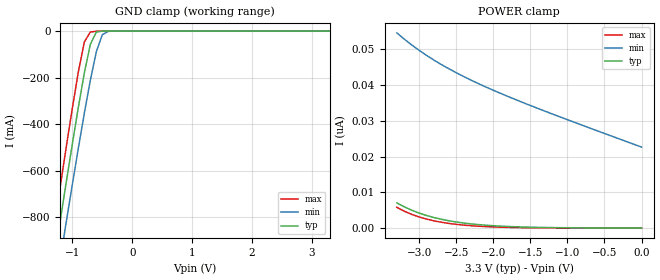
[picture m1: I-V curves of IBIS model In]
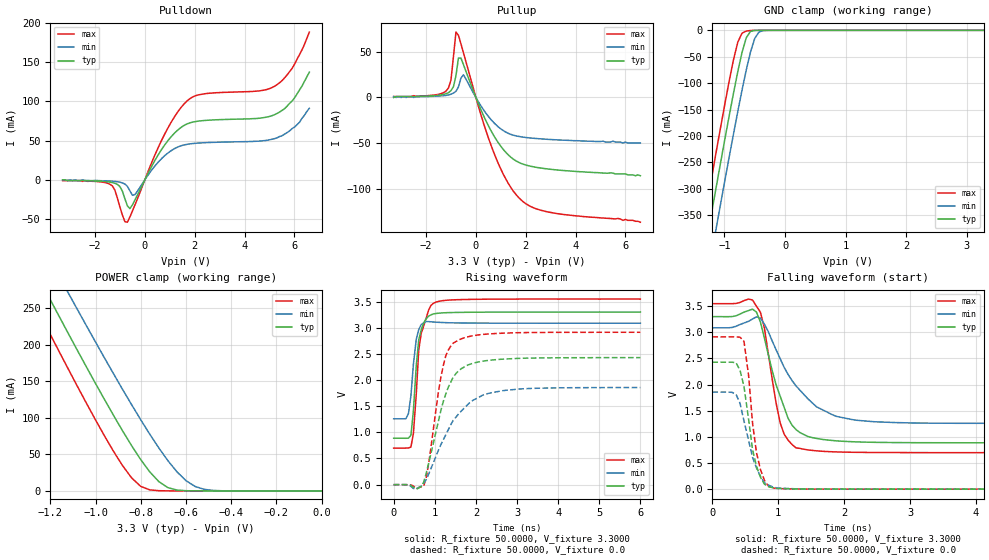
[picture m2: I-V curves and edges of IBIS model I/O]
| IBIS file 71v016.ibs created by s2ibis2 version 1.1
| North Carolina State University Electronics Research Laboratory  1995
[IBIS ver]   2.1
[File name]   71v016.ibs
[File Rev]   3.0
[Date]   Jan 29, 2007
[Source]   HSPICE models at IDT
[Notes]   1. Temperatures: typ=25C, min=100C, max=-40C 2. Cemos11.5 3.3v
   process 3. Ramp rates based on 50ohm load.
[Disclaimer] Integrated Device Technology, Inc. ("IDT") hereby grants the
   user of this IBIS model a non-exclusive, nontransferable
   license to use this IBIS model under the following terms. The
   user is granted this license only to use the IBIS model and is
   not granted rights to sell, copy (except as needed to run the
   IBIS model), rent, lease or sub-license the IBIS model in
   whole or in part, or in modified form to anyone. The User may
   modify the IBIS model to suit its specific applications, but
   rights to derivative works and such modifications shall belong
   to IDT. This IBIS model is provided on an AS IS" basis and IDT
   makes absolutely no warranty with respect to the information
   contained herein. IDT DISCLAIMS AND CUSTOMER WAIVES ALL
   WARRANTIES, EXPRESS AND IMPLIED, INCLUDING WARRANTIES OF
   MERCHANTABILITY AND FITNESS FOR A PARTICULAR PURPOSE. THE
   ENTIRE RISK AS TO QUALITY AND PERFORMANCE IS WITH THE USER
   ACCORDINGLY, IN NO EVENT SHALL IDT BE LIABLE FOR ANY DIRECT OR
   INDIRECT DAMAGES, WHETHER IN CONTRACT OR TORT, INCLUDING ANY
   LOST PROFITS OR OTHER INCIDENTAL, CONSEQUENTIAL, EXEMPLARY, OR
   PUNITIVE DAMAGES ARISING OUT OF THE USE OR APPLICATION OF THE
   IBIS model. Further, IDT reserves the right to make changes
   without notice to any product herein to improve reliability,
   function, or design. IDT does not convey any license under
   patent rights or any other intellectual property rights,
   including those of third parties. IDT is not obligated to
   provide maintenance or support for the licensed IBIS model.
[Copyright]   Copyright 2003, Integrated Device Technology, Inc.
|   Component IDT71V016_PH44 (TSOP 44)
[Component]   IDT71V016_PH44
[Manufacturer]   Integrated Device Technology
[Package]
| variable   typ   min   max
R_pkg   0.1212   0.0774   0.165
L_pkg   5.565nH   3.49nH   7.64nH
C_pkg   0.719pF   0.388pF   1.05pF
[Pin]  signal_name   model_name   R_pin   L_pin   C_pin
| in   in   dummy
| ena  enable   dummy
1   A4   In
2   A3   In
3   A2   In
4   A1   In
5   A0   In
6   CS#   In
7   I/O0   I/O
8   I/O1   I/O
9   I/O2   I/O
10   I/O3   I/O
11   VDD   POWER
12   VSS   GND
13   I/O4   I/O
14   I/O5   I/O
15   I/O6   I/O
16   I/O7   I/O
17   WE#   In
18   A15   In
19   A14   In
20   A13   In
21   A12   In
22   NC   NC
23   NC   NC
24   A11   In
25   A10   In
26   A9   In
27   A8   In
28   NC   NC
29   I/O8   I/O
30   I/O9   I/O
31   I/O10   I/O
32   I/O11   I/O
33   VDD   POWER
34   VSS   GND
35   I/O12   I/O
36   I/O13   I/O
37   I/O14   I/O
38   I/O15   I/O
39   BLE#   In
40   BHE#   In
41   OE#   In
42   A7   In
43   A6   In
44   A5   In
|   Component IDT71V016_PB44 (400 mil SOJ)
[Component]   IDT71V016_PB44
[Manufacturer]   Integrated Device Technology
[Package]
| variable   typ   min   max
R_pkg   0.152   0.099   0.205
L_pkg   7.43nH   3.29nH   11.57nH
C_pkg   1.076pF   0.434pF   1.717pF
[Pin]  signal_name   model_name   R_pin   L_pin   C_pin
| in   in   dummy
| ena  enable   dummy
1   A4   In
2   A3   In
3   A2   In
4   A1   In
5   A0   In
6   CS#   In
7   I/O0   I/O
8   I/O1   I/O
9   I/O2   I/O
10   I/O3   I/O
11   VDD   POWER
12   VSS   GND
13   I/O4   I/O
14   I/O5   I/O
15   I/O6   I/O
16   I/O7   I/O
17   WE#   In
18   A15   In
19   A14   In
20   A13   In
21   A12   In
22   NC   NC
23   NC   NC
24   A11   In
25   A10   In
26   A9   In
27   A8   In
28   NC   NC
29   I/O8   I/O
30   I/O9   I/O
31   I/O10   I/O
32   I/O11   I/O
33   VDD   POWER
34   VSS   GND
35   I/O12   I/O
36   I/O13   I/O
37   I/O14   I/O
38   I/O15   I/O
39   BLE#   In
40   BHE#   In
41   OE#   In
42   A7   In
43   A6   In
44   A5   In
|   Component IDT71V016_BF48
[Component]   IDT71V016_BF48
[Manufacturer]   Integrated Device Technology
[Package]
| variable   typ   min   max
R_pkg   90.00m   75.00m   105.00m
L_pkg   1.85nH   1.50nH   2.20nH
C_pkg   0.35pF   0.30pF   0.40pF
[Pin]  signal_name   model_name   R_pin   L_pin   C_pin
| in   in   dummy
| ena  enable   dummy
A1   BLE#   In
A2   OE#   In
A3   A0   In
A4   A1   In
A5   A2   In
A6   NC   NC
B1   I/O8   I/O
B2   BHE#   In
B3   A3   In
B4   A4   In
B5   CS#   In
B6   I/O0   I/O
C1   I/O9   I/O
C2   I/O10   I/O
C3   A5   In
C4   A6   In
C5   I/O1   I/O
C6   I/O2   I/O
D1   VSS   GND
D2   I/O11   I/O
D3   NC   NC
D4   A7   In
D5   I/O3   I/O
D6   VDD   POWER
E1   VDD   POWER
E2   I/O12   I/O
E3   NC   NC
E4   NC   NC
E5   I/O4   I/O
E6   VSS   GND
F1   I/O14   I/O
F2   I/O13   I/O
F3   A14   In
F4   A15   In
F5   I/O5   I/O
F6   I/O6   I/O
G1   I/O15   I/O
G2   NC   NC
G3   A12   In
G4   A13   In
G5   WE#   In
G6   I/O7   I/O
H1   NC   NC
H2   A8   In
H3   A9   In
H4   A10   In
H5   A11   In
H6   NC   NC
| Models and submodels in the file (2): In (Input), I/O (I/O)
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|   Model In
[Model]   In
Model_type   Input
Vinl =  0.800V
Vinh =  2.000V
C_comp   1.00pF   0.80pF   1.20pF
[Temperature Range]   25.00   100.00   -40.00
[Voltage Range]   3.30V   3.00V   3.60V
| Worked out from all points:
|   GND clamp passes 1 mA (typ) near -0.52 V on its own axis
[GND_clamp]
| voltage   I(typ)   I(min)   I(max)
-3.3V     -4.386A    -4.452A    -4.346A
-1.4V     -1.14A     -1.298A    -1.003A
-1.3V     -973mA     -1.136A    -831mA
-1.2V     -808mA     -975mA     -661mA
-1.1V     -644mA     -815mA     -493mA
-900mV    -326mA     -502mA     -174mA
-800mV    -179mA     -352mA     -46.47mA
-700mV    -57.01mA   -211mA     -4.056mA
-600mV    -4.272mA   -88.62mA   -572uA
-500mV    -177uA     -15.43mA   -49.05uA
-400mV    -6.45uA    -1.057mA   -2.178uA
3.3V      34.49pA    24.98nA    2.972pA
[POWER_clamp]
| Note: Power Clamp current is essentially zero because there is
| no Power Clamp diode on the 71v016h. The chip's Ground Clamp
| diode functions in place of the Power Clamp diode.
| In addition to working to maintain input pin at 0.7 below
| ground at minimum, the Ground Clamp diode also works to
| maintain the input pin at 0.7v above VCC, at maximum, which
| is basically Power Clamp diode's function.
| voltage   I(typ)   I(min)   I(max)
-3.3V     7.071nA    54.64nA    5.834nA
-3.2V     5.969nA    52.89nA    4.754nA
-3.1V     5.03nA     51.27nA    3.866nA
-2.9V     3.552nA    48.35nA    2.543nA
-2.6V     2.081nA    44.62nA    1.337nA
-2.3V     1.203nA    41.43nA    691pA
-1.9V     572pA      37.71nA    279pA
-1.5V     274pA      34.33nA    110pA
0V        34.49pA    22.69nA    4.69pA
|   Model I/O
[Model]   I/O
Model_type   I/O
Polarity   Inverting
Enable   Active-High
Vinl =  0.800V
Vinh =  2.000V
Vmeas =  1.500V
Cref =  5.000pF
Rref =  0.167k
Vref =  1.720V
C_comp   1.00pF   0.80pF   1.20pF
[Temperature Range]   25.00   100.00   -40.00
[Voltage Range]   3.30V   3.00V   3.60V
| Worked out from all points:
|   slope of the pulldown table from 0 to 0.495 V, typ, clamps not added: 16.7 ohm
|   slope of the pullup table from 0 to 0.495 V, typ, clamps not added: 16.1 ohm
|   GND clamp passes 1 mA (typ) near -0.53 V on its own axis
|   POWER clamp passes 1 mA (typ) near -0.63 V on its own axis
|   rising waveform, R_fixture 50.0000, V_fixture 3.3000: 20-80 % time 151ps typ, 134ps min, 200ps max; typ from 0.887 V to 3.3 V
|   rising waveform, R_fixture 50.0000, V_fixture 0.0: 20-80 % time 504ps typ, 804ps min, 341ps max; typ from 0 V to 2.43 V
|   falling waveform, R_fixture 50.0000, V_fixture 3.3000: 20-80 % time 342ps typ, 590ps min, 227ps max; typ from 3.3 V to 0.887 V
|   falling waveform, R_fixture 50.0000, V_fixture 0.0: 20-80 % time 179ps typ, 235ps min, 158ps max; typ from 2.43 V to 0 V
[Pulldown]
| voltage   I(typ)   I(min)   I(max)
-3.3V     0A         0A         -1mA
-1.4V     -2.9mA     -1.6mA     -5.6mA
-1.2V     -4.4mA     -2.1mA     -13.3mA
-1V       -8.6mA     -3mA       -34.7mA
-700mV    -33.2mA    -8.3mA     -53.92mA
-400mV    -25.82mA   -18.97mA   -32.14mA
700mV     39.94mA    27.89mA    52.1mA
1.6V      69.67mA    44.57mA    97.46mA
2.3V      75.25mA    47.07mA    109mA
5.2V      82.8mA     52.4mA     119mA
5.9V      100mA      65mA       141.4mA
6.6V      137mA      91mA       188mA
[Pullup]
|Voltage   I(typ)   I(min)   I(max)
-3.3V     0A         1mA        1mA
-1.2V     4.1mA      2.3mA      7mA
-1V       7.5mA      3.6mA      19.17mA
-800mV    23.97mA    6.85mA     71.84mA
-700mV    43.4mA     11.63mA    68.35mA
-600mV    43.25mA    21.29mA    58.87mA
-500mV    36.14mA    24.83mA    49.17mA
600mV     -36.16mA   -24.06mA   -51.93mA
1.2V      -60.26mA   -38.03mA   -89.54mA
1.7V      -71.02mA   -42.69mA   -109.5mA
2.9V      -78.58mA   -46.01mA   -125.8mA
6.6V      -86mA      -50mA      -137mA
[GND_clamp]
|Voltage   I(typ)   I(min)   I(max)
-3.3V     -1.735A    -1.8A      -1.681A
-1.41V    -474.4mA   -550.9mA   -408.9mA
-1.34V    -428.6mA   -505.6mA   -362.7mA
-1.27V    -383mA     -460.4mA   -316.7mA
-1.2V     -337.7mA   -415.4mA   -271.1mA
-1.13V    -292.7mA   -370.6mA   -225.8mA
-920mV    -160.6mA   -238.6mA   -94.81mA
-780mV    -78.19mA   -153.7mA   -22.29mA
-640mV    -13.93mA   -74.88mA   -1.375mA
-500mV    -218.4uA   -15.26mA   -50.27uA
-360mV    -1.797uA   -481.2uA   -478.1nA
3.28V     34.9pA     1.448uA    2.904pA
[POWER_clamp]
|Voltage   I(typ)   I(min)   I(max)
-3.28V    1.519A     1.539A     1.508A
-1.32V    331.8mA    384.3mA    286.3mA
-1.28V    308.3mA    361.3mA    262.1mA
-1.2V     261.4mA    315.7mA    213.9mA
-1.12V    215mA      270.4mA    166.4mA
-960mV    124.8mA    181.6mA    75.06mA
-840mV    61.72mA    117.7mA    17.69mA
-800mV    42.78mA    97.24mA    6.218mA
-720mV    12.73mA    58.75mA    310.7uA
-600mV    269.3uA    14.07mA    8.809uA
-480mV    2.886uA    682.9uA    240.8nA
0V        35.62pA    27.93nA    4.769pA
[Ramp]
| variable   typ   min   max
dV/dt_r  1.4568/0.5043n   1.1136/0.7941n   1.7478/0.3413n
dV/dt_f  1.4477/0.3422n   1.1400/0.5546n   1.6978/0.2376n
R_load = 50.0000
[Rising Waveform]
R_fixture= 50.0000
V_fixture= 3.3000
|time   V(typ)   V(min)   V(max)
0s        887.2mV    1.259V     698.9mV
300ps     886.6mV    1.262V     699.1mV
420ps     943.2mV    1.697V     719.1mV
480ps     1.41V      2.301V     976.5mV
550ps     2.275V     2.78V      1.731V
610ps     2.769V     2.963V     2.576V
670ps     2.958V     3.061V     2.89V
850ps     3.222V     3.117V     3.337V
970ps     3.264V     3.109V     3.468V
6ns       3.3V       3.086V     3.548V
[Rising Waveform]
R_fixture= 50.0000
V_fixture= 0.0
|time   V(typ)   V(min)   V(max)
0s        0V         0V         0V
550ps     -86.59mV   -73.42mV   -80.64mV
730ps     47.56mV    26.02mV    -28.5mV
850ps     406.5mV    198.1mV    393.1mV
1.15ns    1.423V     767.5mV    2.062V
1.27ns    1.738V     957.3mV    2.469V
1.45ns    2.058V     1.23V      2.705V
1.88ns    2.308V     1.591V     2.84V
2.61ns    2.397V     1.791V     2.894V
6ns       2.428V     1.856V     2.913V
[Falling Waveform]
R_fixture= 50.0000
V_fixture= 3.3000
|time   V(typ)   V(min)   V(max)
0s        3.3V       3.086V     3.548V
610ps     3.443V     3.255V     3.618V
730ps     3.194V     3.272V     3.383V
790ps     2.89V      3.155V     3.081V
1.03ns    1.777V     2.494V     1.267V
1.15ns    1.355V     2.194V     937.4mV
1.27ns    1.14V      1.975V     790mV
1.58ns    970.4mV    1.576V     733.2mV
2.18ns    904.8mV    1.319V     704.9mV
6ns       887.2mV    1.259V     698.9mV
[Falling Waveform]
R_fixture= 50.0000
V_fixture= 0.0
|time   V(typ)   V(min)   V(max)
0s        2.428V     1.856V     2.913V
360ps     2.416V     1.812V     2.914V
420ps     2.275V     1.643V     2.906V
480ps     1.963V     1.305V     2.828V
550ps     1.337V     933.4mV    2.174V
610ps     756.1mV    609.2mV    1.265V
670ps     438.6mV    407.3mV    698.1mV
790ps     96.01mV    123.6mV    170.5mV
910ps     30.18mV    46.54mV    23.43mV
6ns       -10.24uV   22.32uV    15.86uV
